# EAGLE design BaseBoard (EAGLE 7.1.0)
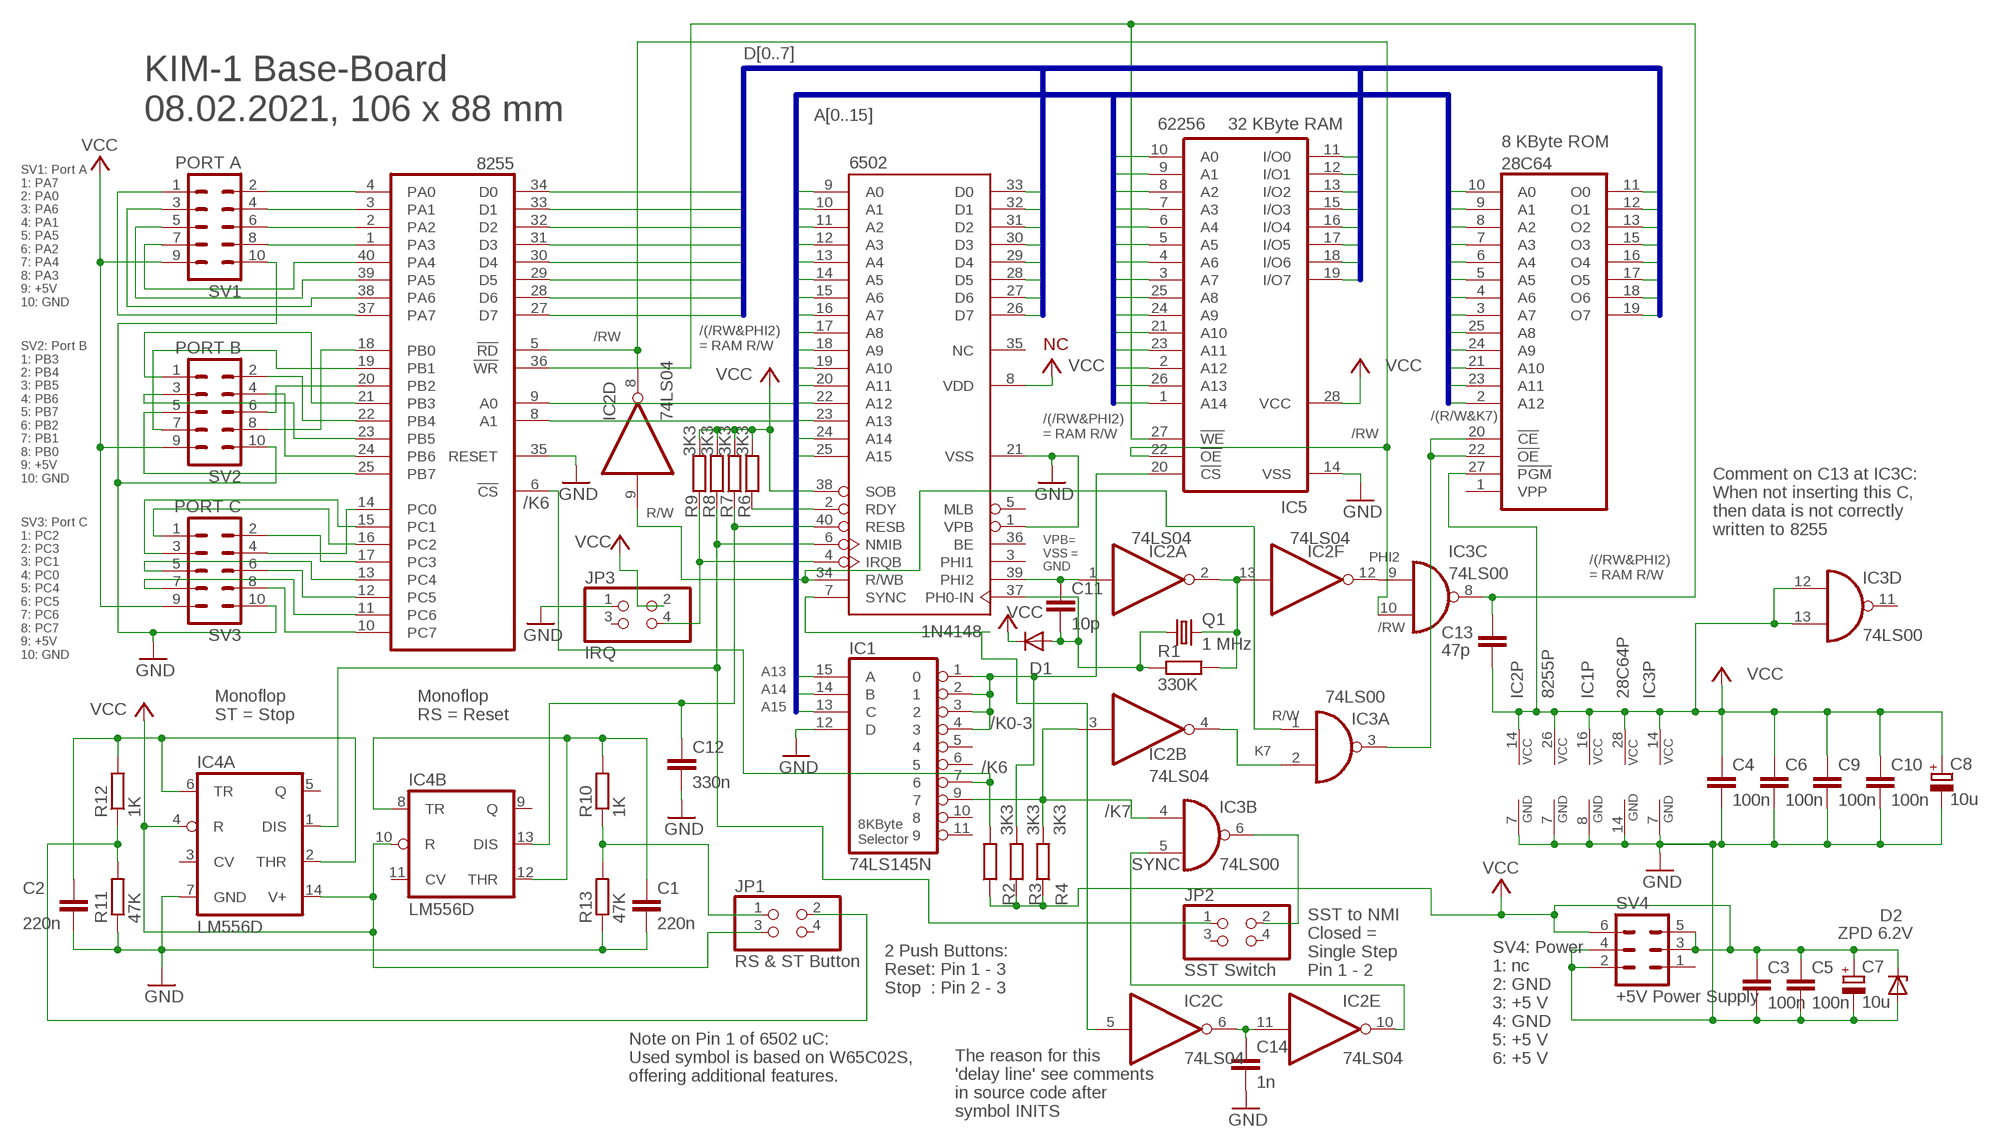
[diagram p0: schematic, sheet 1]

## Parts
28C64  2764  [DIL28]
6502  W65C02SP  [DIP-40]
8255  82C55A  [DIL40]
C1  220n  C-EUC1206  [C1206]
C2  220n  C-EUC1206  [C1206]
C3  100n  C-EUC1206  [C1206]
C4  100n  C-EUC1206  [C1206]
C5  100n  C-EUC1206  [C1206]
C6  100n  C-EUC1206  [C1206]
C7  10u  CPOL-EUE2.5-5  [E2,5-5]
C8  10u  CPOL-EUE2.5-5  [E2,5-5]
C9  100n  C-EUC1206  [C1206]
C10  100n  C-EUC1206  [C1206]
C11  10p  C-EUC1206  [C1206]
C12  330n  C-EUC1206  [C1206]
C13  47p  C-EUC1206  [C1206]
C14  1n  C-EUC1206  [C1206]
D1  1N4148  1N4148DO35-7  [DO35-7]
D2  ZPD 6.2V  ZPD  [DO35Z10]
IC1  74LS145N  [DIL16]
IC2  74LS04  74S04N  [DIL14]
IC3  74LS00  74ALS00N  [DIL14]
IC4  LM556D  [SO14]
IC5  62256  62256P  [DIL28-6]
JP1  RS & ST Button  PINHD-2X2  [2X02]
JP2  SST Switch  PINHD-2X2  [2X02]
JP3  IRQ  PINHD-2X2  [2X02]
Q1  1 MHz  CRYSTALHC18U-V  [HC18U-V]
R1  330K  R-EU_R1206  [R1206]
R2  3K3  R-EU_R1206  [R1206]
R3  3K3  R-EU_R1206  [R1206]
R4  3K3  R-EU_R1206  [R1206]
R6  3K3  R-EU_R1206  [R1206]
R7  3K3  R-EU_R1206  [R1206]
R8  3K3  R-EU_R1206  [R1206]
R9  3K3  R-EU_R1206  [R1206]
R10  1K  R-EU_R1206  [R1206]
R11  47K  R-EU_R1206  [R1206]
R12  1K  R-EU_R1206  [R1206]
R13  47K  R-EU_R1206  [R1206]
SV1  PORT A  ML10  [ML10]
SV2  PORT B  ML10  [ML10]
SV3  PORT C  ML10  [ML10]
SV4  +5V Power Supply  ML6  [ML6]

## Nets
A0: 28C64.10(A0) 6502.9(A0) 8255.9(A0) IC5.10(A0)
A1: 28C64.9(A1) 6502.10(A1) 8255.8(A1) IC5.9(A1)
A2: 28C64.8(A2) 6502.11(A2) IC5.8(A2)
A3: 28C64.7(A3) 6502.12(A3) IC5.7(A3)
A4: 28C64.6(A4) 6502.13(A4) IC5.6(A4)
A5: 28C64.5(A5) 6502.14(A5) IC5.5(A5)
A6: 28C64.4(A6) 6502.15(A6) IC5.4(A6)
A7: 28C64.3(A7) 6502.16(A7) IC5.3(A7)
A8: 28C64.25(A8) 6502.17(A8) IC5.25(A8)
A9: 28C64.24(A9) 6502.18(A9) IC5.24(A9)
A10: 28C64.21(A10) 6502.19(A10) IC5.21(A10)
A11: 28C64.23(A11) 6502.20(A11) IC5.23(A11)
A12: 28C64.2(A12) 6502.22(A12) IC5.2(A12)
A13: 6502.23(A13) IC1.15(A) IC5.26(A13)
A14: 6502.24(A14) IC1.14(B) IC5.1(A14)
A15: 6502.25(A15) IC1.13(C)
D0: 28C64.11(O0) 6502.33(D0) 8255.34(D0) IC5.11(I/O0)
D1: 28C64.12(O1) 6502.32(D1) 8255.33(D1) IC5.12(I/O1)
D2: 28C64.13(O2) 6502.31(D2) 8255.32(D2) IC5.13(I/O2)
D3: 28C64.15(O3) 6502.30(D3) 8255.31(D3) IC5.15(I/O3)
D4: 28C64.16(O4) 6502.29(D4) 8255.30(D4) IC5.16(I/O4)
D5: 28C64.17(O5) 6502.28(D5) 8255.29(D5) IC5.17(I/O5)
D6: 28C64.18(O6) 6502.27(D6) 8255.28(D6) IC5.18(I/O6)
D7: 28C64.19(O7) 6502.26(D7) 8255.27(D7) IC5.19(I/O7)
GND: 28C64.14(GND) 6502.1(VPB) 6502.21(VSS) 8255.7(GND) 8255.35(RESET) C1.2 C2.2 C3.2 C4.2 C5.2 C6.2 C7.- C8.- C9.2 C10.2 C12.2 C14.2 D2.A IC1.8(GND) IC1.12(D) IC2.7(P:GND) IC3.7(P:GND) IC4.7(A:GND) IC5.14(VSS) JP3.1 R11.1 R13.1 SV1.10 SV2.10 SV3.10 SV4.2 SV4.4
N$1: 8255.4(PA0) SV1.2
N$2: 8255.38(PA6) SV1.3
N$3: 8255.3(PA1) SV1.4
N$4: 8255.37(PA7) SV1.1
N$5: 8255.39(PA5) SV1.5
N$6: 8255.2(PA2) SV1.6
N$7: 8255.40(PA4) SV1.7
N$8: 8255.1(PA3) SV1.8
N$9: 6502.7(SYNC) IC2.5(C:I)
N$10: 8255.25(PB7) SV2.5
N$11: 8255.17(PC3) SV3.2
N$12: 8255.16(PC2) SV3.1
N$13: 8255.15(PC1) SV3.3
N$14: 8255.14(PC0) SV3.4
N$15: 8255.13(PC4) SV3.5
N$16: 8255.12(PC5) SV3.6
N$17: 8255.11(PC6) SV3.7
N$18: 8255.10(PC7) SV3.8
N$19: 8255.24(PB6) SV2.4
N$20: 8255.23(PB5) SV2.3
N$21: 8255.22(PB4) SV2.2
N$22: 8255.20(PB2) SV2.6
N$23: 8255.21(PB3) SV2.1
N$24: 8255.19(PB1) SV2.7
N$25: 8255.18(PB0) SV2.8
N$26: IC1.1 IC1.2 IC1.3 IC1.4 IC5.20(!CS) R3.2
N$27: IC1.9 IC2.3(B:I) IC3.4(B:I0) R4.2
N$28: 6502.39(PHI2) C11.1 IC2.1(A:I)
N$29: IC2.2(A:O) IC2.13(F:I) Q1.2 R1.2
N$30: 6502.37(PH0-IN) C11.2 D1.A Q1.1 R1.1
N$31: 8255.5(!RD) IC2.8(D:O) IC3.10(C:I1) IC5.22(!OE)
N$33: 8255.6(!CS) IC1.7 R2.2
N$34: IC2.4(B:O) IC3.2(A:I1)
N$35: 6502.34(R/WB) IC2.9(D:I) IC3.1(A:I0)
N$36: 6502.2(RDY) R6.1
N$37: 28C64.20(!CE) 28C64.22(!OE) IC3.3(A:O)
N$39: 6502.6(NMIB) IC4.1(A:DIS) JP2.1 R8.1
N$40: 6502.4(IRQB) JP3.4 R9.1
N$41: C2.1 IC4.2(A:THR) IC4.6(A:TR) R12.2
N$42: C1.1 IC4.8(B:TR) IC4.12(B:THR) R10.2
N$43: IC3.6(B:O) JP2.2
N$44: JP1.1 R10.1 R13.2
N$46: JP1.2 R11.2 R12.1
N$47: 6502.40(RESB) C12.1 IC4.13(B:DIS) R7.1
N$49: IC2.12(F:O) IC3.9(C:I0)
N$50: 8255.36(!WR) C13.1 IC3.8(C:O) IC5.27(!WE)
N$51: C14.1 IC2.6(C:O) IC2.11(E:I)
N$52: IC2.10(E:O) IC3.5(B:I1)
VCC: 28C64.27(!PGM) 28C64.28(VCC) 6502.8(VDD) 6502.38(SOB) 8255.26(VCC) C3.1 C4.1 C5.1 C6.1 C7.+ C8.+ C9.1 C10.1 C13.2 D1.C D2.C IC1.16(VCC) IC2.14(P:VCC) IC3.12(D:I0) IC3.13(D:I1) IC3.14(P:VCC) IC4.4(A:R) IC4.10(B:R) IC4.14(A:V+) IC5.28(VCC) JP1.3 JP3.2 R2.1 R3.1 R4.1 R6.2 R7.2 R8.2 R9.2 SV1.9 SV2.9 SV3.9 SV4.3 SV4.5 SV4.6
Unconnected: 28C64.1(VPP) 6502.3(PHI1) 6502.5(MLB) 6502.35(NC) 6502.36(BE) IC1.5 IC1.6 IC1.10 IC1.11 IC3.11(D:O) IC4.3(A:CV) IC4.5(A:Q) IC4.9(B:Q) IC4.11(B:CV) JP1.4 JP2.3 JP2.4 JP3.3 SV4.1

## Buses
A[0..15]
D[0..7]

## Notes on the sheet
- KIM-1 Base-Board
  08.02.2021, 106 x 88 mm
- 32 KByte RAM
- 8 KByte ROM
- SV1: Port A
  1: PA7
  2: PA0
  3: PA6
  4: PA1
  5: PA5
  6: PA2
  7: PA4
  8: PA3
  9: +5V
  10: GND
- /RW
- /(/RW&PHI2)
  = RAM R/W
- /(R/W&K7)
- /(/RW&PHI2)
  = RAM R/W
- /RW
- SV2: Port B
  1: PB3
  2: PB4
  3: PB5
  4: PB6
  5: PB7
  6: PB2
  7: PB1
  8: PB0
  9: +5V
  10: GND
- /K6
- R/W
- Comment on C13 at IC3C:
  When not inserting this C,
  then data is not correctly
  written to 8255
- PHI2
- VPB=
  VSS =
  GND
- /(/RW&PHI2)
  = RAM R/W
- /RW
- SV3: Port C
  1: PC2
  2: PC3
  3: PC1
  4: PC0
  5: PC4
  6: PC5
  7: PC6
  8: PC7
  9: +5V
  10: GND
- A13
- A14
- A15
- Monoflop
  ST = Stop
- Monoflop
  RS = Reset
- R/W
- /K0-3
- K7
- /K6
- /K7
- 8KByte
  Selector
- SYNC
- SST to NMI
  Closed =
  Single Step
  Pin 1 - 2
- 2 Push Buttons:
  Reset: Pin 1 - 3
  Stop  : Pin 2 - 3
- SV4: Power
  1: nc
  2: GND
  3: +5 V
  4: GND
  5: +5 V
  6: +5 V
- Note on Pin 1 of 6502 uC:
  Used symbol is based on W65C02S,
  offering additional features.
- The reason for this
  'delay line' see comments
  in source code after
  symbol INITS

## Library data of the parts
28C64 = memory:2764: MEMORY
6502 = 65xxx:W65C02SP: Western Digital Version
8255 = micro-harris:82C55A: MICROCONTROLLER/MEMORY DEVICE; MF: INTERSIL; MPN: CP82C55A-5; OC_FARNELL: 1018158; OC_NEWARK: 06F3290
C1-C6 C9-C14 = rcl:C-EU: CAPACITOR, European symbol
C7 C8 = rcl:CPOL-EU: POLARIZED CAPACITOR, European symbol
D1 = diode:1N4148: DIODE
D2 = diode:ZPD: Z DIODE
IC1 = 74xx-eu:74*145: BCD to decimal DECODER/DRIVER
IC2 = 74xx-eu:74*04: Hex INVERTER
IC3 = 74xx-eu:74*00: Quad 2-input NAND gate
IC4 = linear3:*556: Dual TIMER
IC5 = memory-hitachi:62256P: MEMORY; OC_FARNELL: unknown; OC_NEWARK: unknown
JP1-JP3 = pinhead:PINHD-2X2: PIN HEADER
Q1 = crystal:CRYSTAL: CRYSTAL; OC_FARNELL: unknown; OC_NEWARK: unknown
R1-R4 R6-R13 = rcl:R-EU_: RESISTOR, European symbol
SV1-SV3 = con-harting-ml:ML10: HARTING; OC_FARNELL: unknown; OC_NEWARK: unknown
SV4 = con-harting-ml:ML6: HARTING; OC_FARNELL: unknown; OC_NEWARK: unknown

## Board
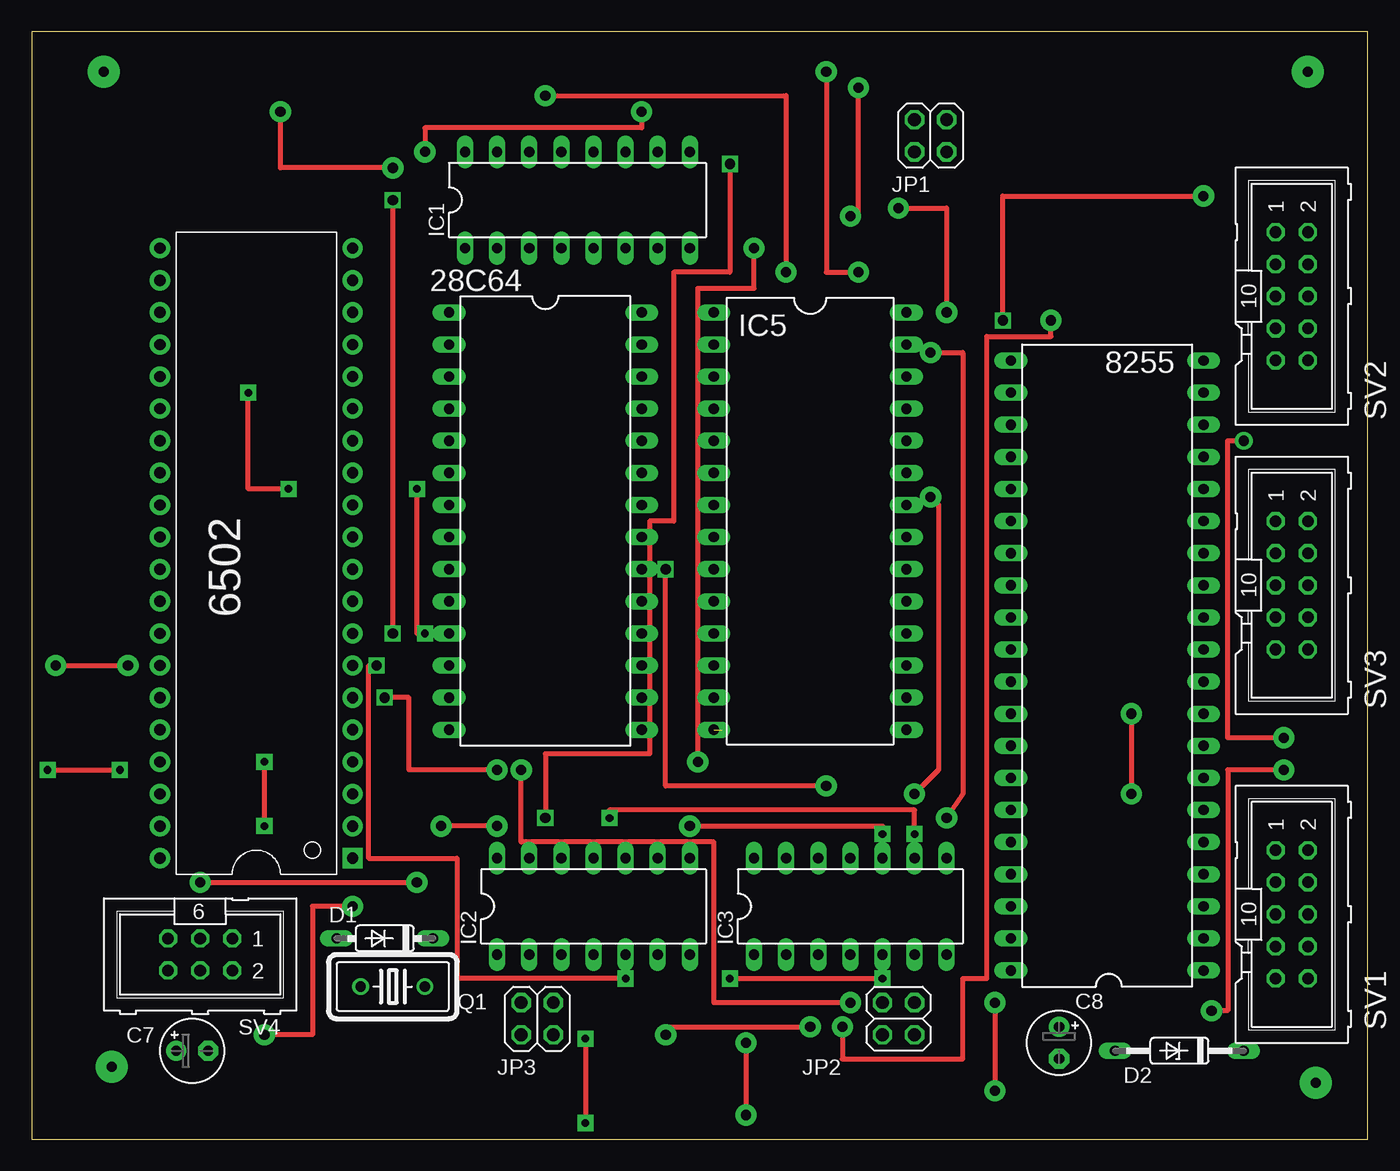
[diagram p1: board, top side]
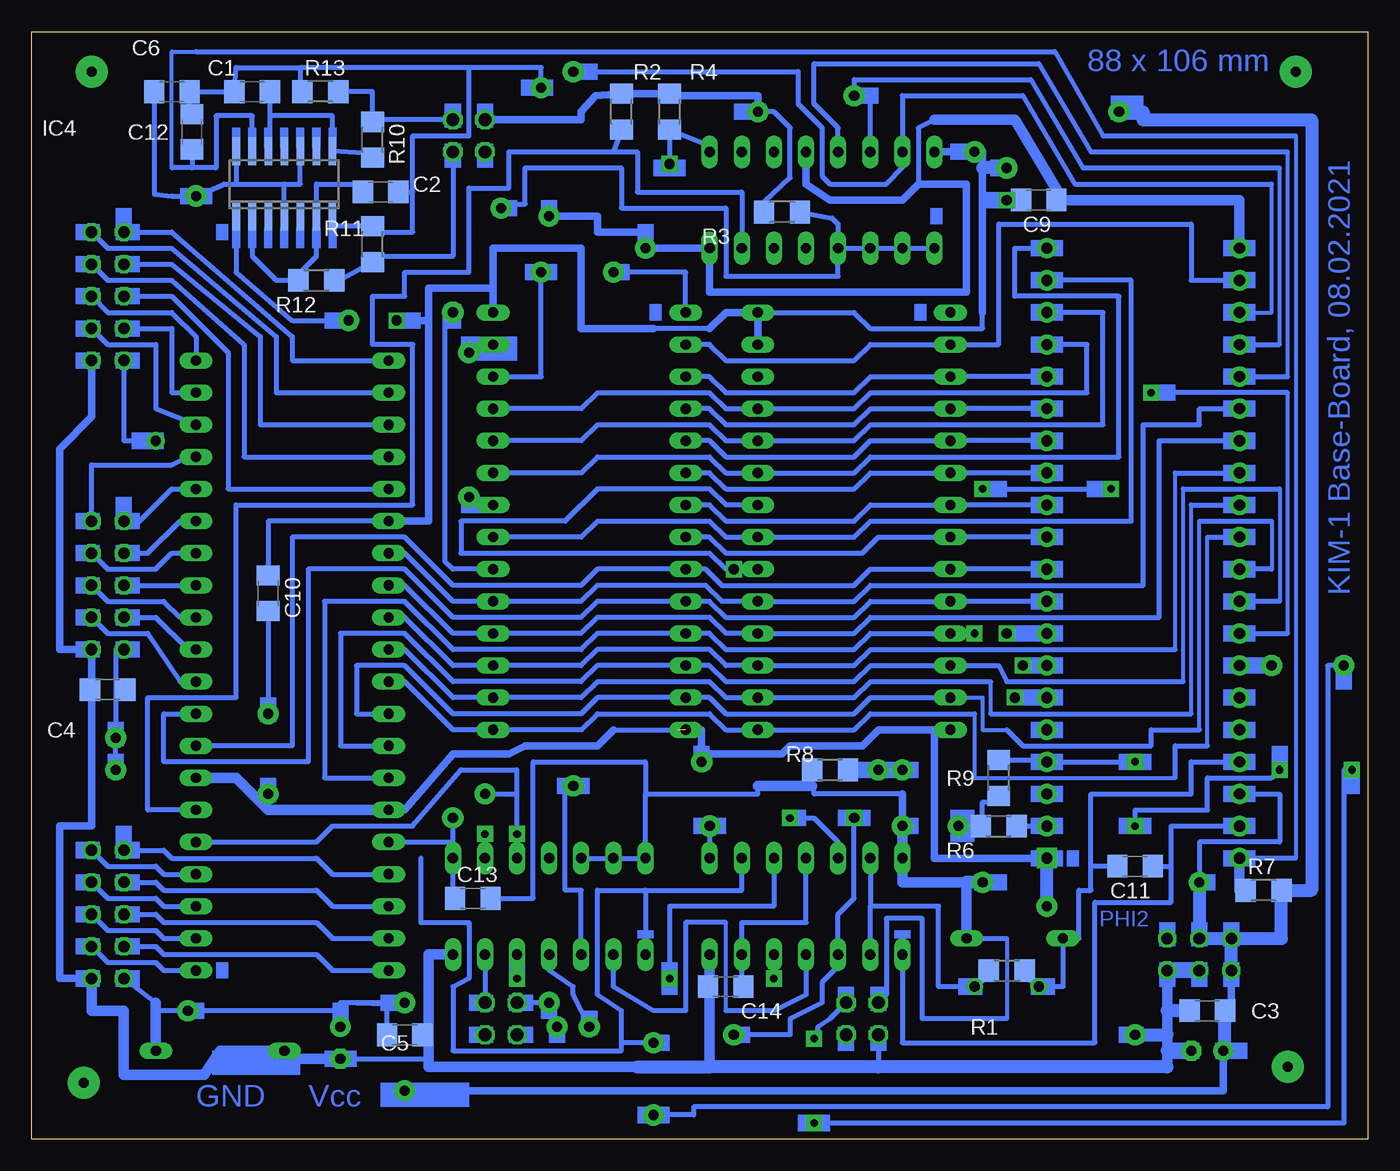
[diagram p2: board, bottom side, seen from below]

Size 105.72 x 87.62 mm. Coordinates in mm from the lower left corner, seen from the top.
Outline: 0,0 105.72,0 105.72,87.62 0,87.62 0,0
Copper layers (1*16): Top 0.035mm / dielectric 1.5mm / Bottom 0.035mm
Design rules "default": minimum track width 10mil, minimum drill 24mil, track to track 8mil, track to pad 8mil, pad to pad 8mil, via to via 8mil, smd to smd 8mil, copper to edge 40mil, drill to drill 8mil, minimum pad ring 10mil, minimum via ring 8mil, stop-mask expansion 4mil, vias tented up to drill 0mil, thermal gap 10mil

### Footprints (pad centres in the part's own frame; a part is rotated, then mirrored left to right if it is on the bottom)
DIL28 = drill 0.813 long: 1 -16.51,-7.62; 2 -13.97,-7.62; 3 -11.43,-7.62; 4 -8.89,-7.62; 5 -6.35,-7.62; 6 -3.81,-7.62; 7 -1.27,-7.62; 8 1.27,-7.62; 9 3.81,-7.62; 10 6.35,-7.62; 11 8.89,-7.62; 12 11.43,-7.62; 13 13.97,-7.62; 14 16.51,-7.62; 15 16.51,7.62; 16 13.97,7.62; 17 11.43,7.62; 18 8.89,7.62; 19 6.35,7.62; 20 3.81,7.62; 21 1.27,7.62; 22 -1.27,7.62; 23 -3.81,7.62; 24 -6.35,7.62; 25 -8.89,7.62; 26 -11.43,7.62; 27 -13.97,7.62; 28 -16.51,7.62
DIP-40 = drill 0.889 pad 1.6 square: 1 -22.86,-7.62 | drill 0.889 pad 1.6: 2 -20.32,-7.62; 3 -17.78,-7.62; 4 -15.24,-7.62; 5 -12.7,-7.62; 6 -10.16,-7.62; 7 -7.62,-7.62; 8 -5.08,-7.62; 9 -2.54,-7.62; 10 0,-7.62; 11 2.54,-7.62; 12 5.08,-7.62; 13 7.62,-7.62; 14 10.16,-7.62; 15 12.7,-7.62; 16 15.24,-7.62; 17 17.78,-7.62; 18 20.32,-7.62; 19 22.86,-7.62; 20 25.4,-7.62; 21 25.4,7.62; 22 22.86,7.62; 23 20.32,7.62; 24 17.78,7.62; 25 15.24,7.62; 26 12.7,7.62; 27 10.16,7.62; 28 7.62,7.62; 29 5.08,7.62; 30 2.54,7.62; 31 0,7.62; 32 -2.54,7.62; 33 -5.08,7.62; 34 -7.62,7.62; 35 -10.16,7.62; 36 -12.7,7.62; 37 -15.24,7.62; 38 -17.78,7.62; 39 -20.32,7.62; 40 -22.86,7.62
DIL40 = drill 0.813 long: 1 -24.13,-7.62; 2 -21.59,-7.62; 3 -19.05,-7.62; 4 -16.51,-7.62; 5 -13.97,-7.62; 6 -11.43,-7.62; 7 -8.89,-7.62; 8 -6.35,-7.62; 9 -3.81,-7.62; 10 -1.27,-7.62; 11 1.27,-7.62; 12 3.81,-7.62; 13 6.35,-7.62; 14 8.89,-7.62; 15 11.43,-7.62; 16 13.97,-7.62; 17 16.51,-7.62; 18 19.05,-7.62; 19 21.59,-7.62; 20 24.13,-7.62; 21 24.13,7.62; 22 21.59,7.62; 23 19.05,7.62; 24 16.51,7.62; 25 13.97,7.62; 26 11.43,7.62; 27 8.89,7.62; 28 6.35,7.62; 29 3.81,7.62; 30 1.27,7.62; 31 -1.27,7.62; 32 -3.81,7.62; 33 -6.35,7.62; 34 -8.89,7.62; 35 -11.43,7.62; 36 -13.97,7.62; 37 -16.51,7.62; 38 -19.05,7.62; 39 -21.59,7.62; 40 -24.13,7.62
C1206 = smd 1.6 x 1.8: 1 -1.4,0; 2 1.4,0
E2,5-5 = drill 0.813 pad 1.6: + -1.27,0 | drill 0.813 pad 1.6 octagon: - 1.27,0
DO35-7 = drill 0.813 long: A 3.81,0; C -3.81,0
DO35Z10 = drill 0.813 long: A 5.08,0; C -5.08,0
DIL16 = drill 0.813 long: 1 -8.89,-3.81; 2 -6.35,-3.81; 3 -3.81,-3.81; 4 -1.27,-3.81; 5 1.27,-3.81; 6 3.81,-3.81; 7 6.35,-3.81; 8 8.89,-3.81; 9 8.89,3.81; 10 6.35,3.81; 11 3.81,3.81; 12 1.27,3.81; 13 -1.27,3.81; 14 -3.81,3.81; 15 -6.35,3.81; 16 -8.89,3.81
DIL14 = drill 0.813 long: 1 -7.62,-3.81; 2 -5.08,-3.81; 3 -2.54,-3.81; 4 0,-3.81; 5 2.54,-3.81; 6 5.08,-3.81; 7 7.62,-3.81; 8 7.62,3.81; 9 5.08,3.81; 10 2.54,3.81; 11 0,3.81; 12 -2.54,3.81; 13 -5.08,3.81; 14 -7.62,3.81
SO14 = smd 0.6 x 2.2: 1 -3.81,-2.6; 2 -2.54,-2.6; 3 -1.27,-2.6; 4 0,-2.6; 5 1.27,-2.6; 6 2.54,-2.6; 7 3.81,-2.6; 8 3.81,2.6; 9 2.54,2.6; 10 1.27,2.6; 11 0,2.6; 12 -1.27,2.6; 13 -2.54,2.6; 14 -3.81,2.6
DIL28-6 = drill 0.813 long: 1 -16.51,-7.62; 2 -13.97,-7.62; 3 -11.43,-7.62; 4 -8.89,-7.62; 5 -6.35,-7.62; 6 -3.81,-7.62; 7 -1.27,-7.62; 8 1.27,-7.62; 9 3.81,-7.62; 10 6.35,-7.62; 11 8.89,-7.62; 12 11.43,-7.62; 13 13.97,-7.62; 14 16.51,-7.62; 15 16.51,7.62; 16 13.97,7.62; 17 11.43,7.62; 18 8.89,7.62; 19 6.35,7.62; 20 3.81,7.62; 21 1.27,7.62; 22 -1.27,7.62; 23 -3.81,7.62; 24 -6.35,7.62; 25 -8.89,7.62; 26 -11.43,7.62; 27 -13.97,7.62; 28 -16.51,7.62
2X02 = drill 1.016 octagon: 1 -1.27,-1.27; 2 -1.27,1.27; 3 1.27,-1.27; 4 1.27,1.27
HC18U-V = drill 0.813: 1 -2.54,0; 2 2.54,0
R1206 = smd 1.6 x 1.803: 1 -1.422,0; 2 1.422,0
ML10 = drill 0.914 octagon: 1 -5.08,-1.27; 2 -5.08,1.27; 3 -2.54,-1.27; 4 -2.54,1.27; 5 0,-1.27; 6 0,1.27; 7 2.54,-1.27; 8 2.54,1.27; 9 5.08,-1.27; 10 5.08,1.27
ML6 = drill 0.914 octagon: 1 -2.54,-1.27; 2 -2.54,1.27; 3 0,-1.27; 4 0,1.27; 5 2.54,-1.27; 6 2.54,1.27

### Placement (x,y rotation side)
28C64  40.64,48.9 270 top
6502  17.78,45.09 90 top
8255  85.09,37.47 90 top
C1  88.27,82.87 180 bottom
C2  78.11,74.93 0 bottom
C3  12.7,10.16 180 bottom
C4  99.7,35.56 180 bottom
C5  76.2,8.26 0 bottom
C6  94.62,82.87 0 bottom
C7  12.7,6.99 0 top
C8  81.28,7.62 270 top
C9  26.04,74.29 0 bottom
C10  87,43.18 270 bottom
C11  18.41,21.59 180 bottom
C12  93.03,79.69 90 bottom
C13  70.8,19.05 0 bottom
C14  50.8,12.07 180 bottom
D1  27.94,15.88 180 top
D2  90.81,6.99 180 top
IC1  43.18,74.29 0 top
IC2  44.45,18.41 0 top
IC3  64.77,18.41 0 top
IC4  85.73,75.56 0 bottom
IC5  61.59,48.9 270 top
JP1  71.12,79.38 180 top
JP2  68.58,9.53 270 top
JP3  40.01,9.53 0 top
Q1  28.57,12.07 0 top
R1  28.57,13.34 180 bottom
R2  59.05,81.28 270 bottom
R3  46.36,73.34 0 bottom
R4  55.25,81.28 270 bottom
R6  29.21,24.77 180 bottom
R7  8.26,19.69 0 bottom
R8  42.55,29.21 180 bottom
R9  29.21,28.57 270 bottom
R10  78.74,79.06 270 bottom
R11  78.74,70.8 270 bottom
R12  83.19,67.94 180 bottom
R13  82.87,82.87 0 bottom
SV1  99.7,17.78 270 top
SV2  99.7,66.67 270 top
SV3  99.7,43.81 270 top
SV4  13.34,14.61 180 top

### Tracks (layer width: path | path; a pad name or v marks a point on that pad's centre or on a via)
A0
  Bottom 0.406: 6502.9 28C64.10 39.37,42.55 40.64,41.27 50.8,41.27 52.07,42.55 IC5.10 60.96,42.55 62.23,41.27 72.39,41.27 76.2,45.09 83.82,45.09 83.82,29.84 95.25,29.84 95.25,33.66 8255.9
A1
  Bottom 0.406: 6502.10 28C64.9 39.37,45.09 40.64,43.81 51.12,43.81 52.39,45.09 IC5.9 60.96,45.09 62.23,43.81 72.39,43.81 76.2,47.62 85.09,47.62 85.09,31.12 8255.8
A2
  Bottom 0.406: 6502.11 28C64.8 38.73,47.62 40.01,46.35 50.8,46.35 52.07,47.62 IC5.8
A3
  Bottom 0.406: 6502.12 28C64.7 39.37,50.16 40.64,48.9 50.8,48.9 52.07,50.16 IC5.7
A4
  Bottom 0.406: 6502.13 28C64.6 39.37,52.7 40.64,51.44 50.8,51.44 52.07,52.7 IC5.6
A5
  Bottom 0.406: 6502.14 28C64.5 39.37,55.24 40.64,53.98 50.8,53.98 52.07,55.24 IC5.5
A6
  Bottom 0.406: 6502.15 28C64.4 39.37,57.79 40.64,56.52 50.8,56.52 52.07,57.79 IC5.4
A7
  Bottom 0.406: 6502.16 28C64.3 39.37,60.33 40.64,59.05 50.8,59.05 52.07,60.33 IC5.3
A8
  Bottom 0.406: 6502.17 22.22,62.87 22.22,59.05 39.37,59.05 40.64,57.79 28C64.25 50.8,57.79 52.07,59.05 60.96,59.05 62.23,57.79 IC5.25
A9
  Bottom 0.406: 6502.18 20.95,65.41 20.95,56.52 39.37,56.52 40.64,55.24 28C64.24 50.8,55.24 52.07,56.52 60.96,56.52 62.23,55.24 IC5.24
A10
  Bottom 0.406: 6502.19 18.73,67.94 18.73,48.9 39.37,48.9 40.64,47.62 28C64.21 50.8,47.62 52.07,48.9 60.96,48.9 62.23,47.62 IC5.21
A11
  Bottom 0.406: 6502.20 27.94,70.49 27.94,66.67 19.68,66.67 19.68,53.98 39.37,53.98 40.64,52.7 28C64.23 50.8,52.7 52.07,53.98 60.96,53.98 62.23,52.7 IC5.23
A12
  Bottom 0.406: 6502.22 13.97,67.94 13.97,72.39 29.21,72.39 29.21,62.87 28C64.2 39.37,62.87 40.64,61.59 50.8,61.59 52.07,62.87 IC5.2
A13  (via drill 0.8 pad 1.68)
  Top 0.406: v62.87,84.46 62.87,68.58 v65.41,68.58
  Bottom 0.305: 6502.23 7.62,65.41 7.62,75.56
  Bottom 0.406: 7.62,75.56 23.18,75.56 27.3,82.55 36.83,82.55 IC1.15 36.83,76.84 38.1,75.56 42.55,75.56 43.18,76.2 43.18,80.01 45.09,81.91 45.09,84.46 v62.87,84.46 | IC5.26 65.41,60.33 v65.41,68.58
A14  (via drill 0.8 pad 1.68)
  Top 0.406: v40.64,82.55 59.69,82.55 v59.69,68.58
  Bottom 0.305: 6.98,62.87 6.98,76.84
  Bottom 0.406: 6502.24 6.98,62.87 | IC1.14 39.37,82.55 v40.64,82.55 40.64,83.82 26.67,83.82 22.54,76.84 6.98,76.84 | IC5.1 53.98,68.58 v59.69,68.58
A15
  Bottom 0.305: 6.35,60.33 6.35,78.1
  Bottom 0.406: 6502.25 6.35,60.33 | IC1.13 41.91,80.01 43.82,81.91 43.82,85.09 26.04,85.09 21.91,78.1 6.35,78.1
D0  (via drill 0.6 pad 1.27)
  Top 0.406: v31.11,40.01 30.48,40.01 v30.48,51.44 | v20.32,51.44 17.14,51.44 v17.14,59.05
  Bottom 0.305: 6.35,40.01 6.35,59.05
  Bottom 0.406: 8255.34 82.55,28.57 82.55,42.55 76.2,42.55 72.39,38.73 62.23,38.73 60.96,40.01 IC5.11 52.07,40.01 50.8,38.73 40.64,38.73 39.37,40.01 28C64.11 v31.11,40.01 | 6502.33 6.35,40.01 | 6.35,59.05 v17.14,59.05 | v30.48,51.44 v20.32,51.44
D1
  Bottom 0.305: 14.61,36.2 14.61,51.44 | 6.98,51.44 6.98,42.55
  Bottom 0.406: 14.61,36.2 28.57,36.2 29.21,37.47 28C64.12 39.37,37.47 40.64,36.2 50.8,36.2 52.07,37.47 IC5.12 60.96,37.47 62.23,36.2 72.39,36.2 76.2,40.01 81.28,40.01 81.28,31.12 8255.33 | 14.61,51.44 6.98,51.44 | 6.98,42.55 6502.32
D2
  Bottom 0.305: 28C64.13 30.48,34.92 30.48,32.39 28.57,32.39 | 13.34,32.39 13.34,48.9 | 7.62,48.9 7.62,45.09
  Bottom 0.406: 28C64.13 39.37,34.92 40.64,33.66 50.8,33.66 52.07,34.92 IC5.13 60.96,34.92 62.23,33.66 72.39,33.66 76.2,37.47 80.01,37.47 80.01,33.66 8255.32 | 28.57,32.39 27.3,31.12 17.14,31.12 17.14,32.39 13.34,32.39 | 13.34,48.9 7.62,48.9 | 7.62,45.09 6502.31
D3
  Bottom 0.305: 31.11,33.66 31.11,28.57 15.24,28.57 | 12.7,31.12 12.7,47.62
  Bottom 0.406: 8255.31 76.2,36.2 72.39,32.39 IC5.15 62.23,32.39 60.96,33.66 52.07,33.66 50.8,32.39 28C64.15 40.64,32.39 39.37,33.66 31.11,33.66 | 15.24,28.57 15.24,31.12 12.7,31.12 | 12.7,47.62 6502.30
D4
  Bottom 0.305: 29.84,36.2 29.84,33.66 | 13.97,33.66 13.97,50.16
  Bottom 0.406: 8255.30 76.2,38.73 72.39,34.92 IC5.16 62.23,34.92 60.96,36.2 52.07,36.2 50.8,34.92 28C64.16 40.64,34.92 39.37,36.2 29.84,36.2 | 29.84,33.66 13.97,33.66 | 13.97,50.16 6502.29
D5
  Bottom 0.305: 15.24,38.73 15.24,52.7
  Bottom 0.406: 8255.29 76.2,41.27 72.39,37.47 IC5.17 62.23,37.47 60.96,38.73 52.07,38.73 50.8,37.47 28C64.17 40.64,37.47 39.37,38.73 15.24,38.73 | 15.24,52.7 6502.28
D6
  Bottom 0.406: 8255.28 76.2,43.81 72.39,40.01 IC5.18 62.23,40.01 60.96,41.27 52.07,41.27 50.8,40.01 28C64.18 40.64,40.01 39.37,41.27 16.51,41.27 16.51,55.24 6502.27
D7
  Bottom 0.406: 8255.27 76.2,46.35 72.39,42.55 IC5.19 62.23,42.55 60.96,43.81 52.39,43.81 51.12,42.55 28C64.19 40.64,42.55 39.37,43.81 17.78,43.81 17.78,56.52 13.34,56.52 13.34,57.79 6502.26
GND  (via drill 0.8 pad 1.68)  (1 unrouted)
  Top 0.406: v52.71,29.84 52.71,67.31 57.15,67.31 v57.15,70.49 | v64.77,73.03 65.41,73.03 v65.41,83.19 | v25.4,18.41 22.22,18.41 22.22,8.26 v18.41,8.26 | v87,33.66 v87,27.3
  Bottom 0.406: 34.29,32.39 28C64.14 | 34.29,80.65 35.56,80.01 35.56,75.56 | 8255.35 76.2,26.04 | 84.45,84.77 89.53,84.77 89.67,83.06 C1.2 C6.2 93.22,81.09 C12.2 | 84.45,84.77 84.45,82.4 R13.1 | IC4.7 81.92,72.22 R11.1 78.74,71.75 75.56,71.75 75.56,74.93 | 75.56,74.93 75.56,79.38 71.12,79.38 71.12,84.77 | 71.12,84.77 84.45,84.77 | C2.2 75.56,74.93 | v65.41,83.19 65.41,84.77 71.12,84.77 | C5.2 74.3,8.26 | C8.- 74.3,6.35 | C4.2 100.97,35.56 | 59.69,32.39 54.61,32.39 | C9.2 24.3,74.29 24.3,74.57 | C10.2 v87,33.66 | v87,27.3 87,26.04 | JP3.1 38.73,5.71 | C14.2 52.07,12.07 IC2.7
  Bottom 0.61: 28C64.14 38.73,32.39 40.01,31.12 45.72,31.12 46.36,30.48 52.71,30.48 | 52.71,30.48 52.71,32.39 IC5.14 | 76.2,26.04 72.39,30.48 67.95,30.48 66.67,31.12 60.96,31.12 59.69,32.39 | 6502.1 34.29,22.23 34.29,32.39 | v52.71,29.84 52.71,30.48 | IC1.12 44.45,75.56 42.55,74.29 36.83,74.29 35.56,75.56 31.75,75.56 31.75,66.99 52.07,66.99 IC1.8 v57.15,70.49 57.15,71.75 60.96,71.75 60.96,73.03 v64.77,73.03 | SV2.10 100.97,57.15 103.5,54.61 103.5,38.73 SV3.10 100.97,35.56 100.97,24.77 103.5,24.77 103.5,12.7 SV1.10
  Bottom 0.813: 8255.7 89.53,28.57 87,26.04 8255.35 | 6502.21 10.16,74.29 24.13,74.29 24.3,74.57 27.94,80.65 34.29,80.65 | IC3.7 74.3,14.61 74.3,8.26 74.3,6.35 74.3,5.71 57.79,5.71 | 52.07,5.71 IC2.7 | SV4.2 15.88,10.16 15.88,8.26 15.88,6.99 15.88,5.71 | C8.- 85.73,6.35 D2.A 90.81,6.99 92.08,5.08 98.42,5.08 98.42,10.16 100.97,10.16 SV1.10
  Bottom 1.016: 57.79,5.71 52.07,5.71 38.73,5.71 15.88,5.71 | C3.2 15.88,10.16 | v18.41,8.26 15.88,8.26 | v25.4,18.41 6502.1 | C7.- 15.88,6.99
  Bottom 1.27: SV4.4 SV4.2
N$1
  Bottom 0.406: SV1.2 99.7,21.59 95.89,21.59 95.25,20.96 8255.4
N$2
  Bottom 0.406: SV1.3 95.89,20.32 95.25,19.69 83.19,19.69 81.92,18.41 8255.38
N$3
  Bottom 0.406: SV1.4 99.7,19.05 95.89,19.05 95.25,18.41 8255.3
N$4
  Bottom 0.406: SV1.1 95.25,22.86 94.62,22.23 83.19,22.23 81.92,20.96 8255.37
N$5
  Bottom 0.406: SV1.5 95.89,17.78 95.25,17.14 83.19,17.14 81.92,15.88 8255.39
N$6
  Bottom 0.406: SV1.6 99.7,16.51 95.89,16.51 95.25,15.88 8255.2
N$7
  Bottom 0.406: SV1.7 95.89,15.24 95.25,14.61 83.19,14.61 81.92,13.34 8255.40
N$8
  Bottom 0.406: SV1.8 99.7,13.97 95.89,13.97 95.25,13.34 8255.1
N$9  (via drill 0.6 pad 1.27, 0.8 pad 1.27)
  Top 0.406: v27.3,37.47 26.67,37.47 26.67,22.23 33.66,22.23 33.66,12.7 v46.99,12.7
  Bottom 0.406: v27.3,37.47 6502.7 | IC2.5 v46.99,12.7
N$10
  Bottom 0.406: SV2.5 94.62,66.67 90.17,62.23 90.17,51.44 8255.25
N$11
  Bottom 0.406: SV3.2 100.97,53.34 94.62,53.34 93.34,53.98 8255.17
N$12
  Bottom 0.406: SV3.1 97.16,48.9 94.62,51.44 8255.16
N$13
  Bottom 0.406: SV3.3 96.52,46.35 93.98,48.9 8255.15
N$14
  Bottom 0.406: SV3.4 99.7,45.09 95.89,45.09 94.62,46.35 8255.14
N$15
  Bottom 0.406: SV3.5 8255.13
N$16
  Bottom 0.406: SV3.6 99.7,42.55 95.25,42.55 93.98,41.27 8255.12
N$17
  Bottom 0.406: SV3.7 95.89,41.27 93.34,38.73 8255.11
N$18
  Bottom 0.406: SV3.8 99.7,40.01 96.52,40.01 93.98,36.2 8255.10
N$19
  Bottom 0.406: SV2.4 99.7,67.94 94.62,67.94 88.9,62.87 88.9,53.98 8255.24
N$20
  Bottom 0.406: SV2.3 94.62,69.22 87.63,63.5 87.63,56.52 8255.23
N$21
  Bottom 0.406: SV2.2 99.7,70.49 94.62,70.49 86.36,63.5 86.36,59.05 8255.22
N$22
  Bottom 0.406: SV2.6 99.7,65.41 94.62,65.41 92.71,63.5 8255.20
N$23
  Bottom 0.406: SV2.1 94.62,71.75 85.09,63.5 85.09,61.59 8255.21
N$24
  Bottom 0.406: SV2.7 94.62,64.13 94.62,59.05 8255.19
N$25
  Bottom 0.406: SV2.8 99.7,62.87 95.89,62.87 95.89,57.79 8255.18
N$26  (via drill 0.8 pad 1.68)
  Top 0.406: v68.58,73.66 72.39,73.66 v72.39,65.41
  Bottom 0.406: v68.58,73.66 68.58,73.98 66.67,73.98 66.67,76.84 59.05,76.84 59.05,73.66 50.8,73.66 50.8,68.26 41.91,68.26 IC1.4 | IC1.4 IC1.3 IC1.2 IC1.1 34.14,70.64 34.29,70.64 | IC5.20 72.39,45.09 73.03,45.72 73.03,65.41 v72.39,65.41 | R3.2 42.39,72.87 41.91,72.39 IC1.4
N$27  (via drill 0.8 pad 1.27, 0.8 pad 1.68)
  Top 0.406: v50.16,8.26 50.16,8.89 v61.59,8.89 | v55.25,77.15 55.25,68.58 50.8,68.58 50.8,48.9 48.9,48.9 48.9,30.48 40.64,30.48 v40.64,25.4
  Bottom 0.406: v50.16,8.26 45.72,8.26 45.72,9.53 43.18,10.79 43.18,12.38 41.91,13.65 IC2.3 41.91,17.78 40.64,19.05 v40.64,25.4 | v61.59,8.89 62.87,11.43 62.87,12.07 64.77,13.34 IC3.4 | IC1.9 52.07,78.59 R4.2 v55.25,77.15
N$28
  Bottom 0.406: IC2.1 36.83,7.62 21.59,7.62 21.59,18.73 15.56,18.73 15.56,21.59 | 15.56,21.59 15.56,24.77 6502.39 | C11.1 15.56,21.59
N$29
  Bottom 0.406: R1.2 30,12.85 Q1.2 33.97,12.07 33.97,18.41 39.37,18.41 | IC2.2 39.37,18.41 | IC2.13 39.37,18.41
N$30
  Bottom 0.406: 21.91,21.59 21.91,19.69 22.86,19.69 22.86,15.88 D1.A 24.13,12.07 Q1.1 27.15,12.85 R1.1 | 21.91,21.59 21.91,27.3 13.97,27.3 13.97,29.84 6502.37 | C11.2 21.91,21.59
N$31  (via drill 0.6 pad 1.27, 0.8 pad 1.68)
  Top 0.406: v52.07,24.77 67.31,24.77 v67.31,24.13 | v69.85,27.3 71.75,29.21 71.75,50.16 v71.12,50.8
  Bottom 0.406: 8255.5 83.19,23.5 81.92,24.77 75.56,24.77 71.75,29.21 67.31,29.21 67.31,27.3 | IC3.10 v67.31,24.13 67.31,27.3 | v52.07,24.77 IC2.8 | v69.85,27.3 67.31,27.3 | IC5.22 70.48,50.16 v71.12,50.8
N$32  (via drill 0.8 pad 2.54)
  other vias: 5.71,84.46
N$33
  Bottom 0.406: 59.69,78.1 67.95,78.1 67.95,75.25 71.12,75.25 71.12,68.58 76.2,68.58 76.2,66.67 78.74,66.67 78.74,62.87 75.56,62.87 75.56,50.16 89.53,50.16 89.53,34.92 96.52,34.92 96.52,26.04 8255.6 | 59.69,78.1 57.79,78.1 57.79,74.93 49.53,74.93 IC1.7 | R2.2 59.69,78.1
N$34
  Bottom 0.305: 50.8,10.16 50.8,17.14
  Bottom 0.406: IC2.4 44.45,11.43 46.99,10.16 50.8,10.16 | 50.8,17.14 53.98,17.14 53.98,10.16 56.52,10.16 59.69,12.07 IC3.2
N$35  (via drill 0.8 pad 1.68)
  Top 0.406: v56.52,7.62 v56.52,1.91 | v1.91,37.47 v7.62,37.47
  Bottom 0.406: 74.93,22.23 74.93,17.14 71.12,17.14 71.12,12.7 72.39,12.07 72.39,6.99 59.05,6.99 59.05,7.62 | 59.05,7.62 59.05,10.16 60.96,11.43 60.96,19.69 57.15,19.69 | 57.15,19.69 IC3.1 | 57.15,19.69 49.53,19.69 IC2.9 | v7.62,37.47 6502.34 | v56.52,7.62 59.05,7.62 | v1.91,37.47 3.17,37.47 3.17,2.54 53.34,2.54 53.34,1.91 v56.52,1.91
N$36
  Bottom 0.406: R6.1 6502.2
N$37  (via drill 0.8 pad 1.27, 0.8 pad 1.68)
  Top 0.406: v62.87,27.94 50.16,27.94 v50.16,45.09
  Bottom 0.406: 28C64.20 v50.16,45.09 50.8,45.09 52.07,46.35 71.75,46.35 71.75,48.9 63.5,48.9 60.96,51.44 52.07,51.44 50.8,50.16 28C64.22 | IC3.3 62.23,19.69 63.5,19.69 63.5,27.3 v62.87,27.94
N$38  (via drill 0.8 pad 2.54)
  other vias: 100.97,84.46
N$39  (via drill 0.8 pad 1.27, 0.8 pad 1.68)
  Top 0.406: v36.83,29.21 29.84,29.21 29.84,34.92 v27.94,34.92 | v64.77,10.79 53.98,10.79 53.98,23.5 38.73,23.5 v38.73,29.21 | v64.14,8.89 64.14,6.35 73.66,6.35 73.66,12.7 75.56,12.7 75.56,63.5 80.64,63.5 v80.64,64.77
  Bottom 0.406: 6502.6 v27.94,34.92 | JP2.1 v64.77,10.79 v64.14,8.89 | v36.83,29.21 v38.73,29.21 R8.1 | IC4.1 89.53,68.58 85.09,64.77 v80.64,64.77
N$40  (via drill 0.6 pad 1.27)
  Top 0.406: v18.41,29.84 v18.41,24.77 | v1.27,29.21 v6.98,29.21 | v43.82,7.94 v43.82,1.27
  Bottom 0.406: R9.1 25.55,30 6502.4 v18.41,29.84 | v18.41,24.77 18.41,26.04 12.7,26.04 12.7,28.57 7.62,28.57 v6.98,29.21 | v43.82,7.94 43.5,8.57 43.5,8.89 42.55,9.53 JP3.4 | v1.27,29.21 1.91,29.21 1.91,1.27 v43.82,1.27
N$41
  Bottom 0.406: 84.45,67.79 R12.2 | R12.2 84.61,68.43 83.19,69.85 IC4.6 83.19,75.56 80.01,75.56 80.01,74.93 C2.1 79.38,74.93 | IC4.2 88.27,69.85 86.36,67.94 R12.2
N$42
  Bottom 0.406: R10.2 78.84,77.95 IC4.8 | C1.1 86.87,80.96 | 86.87,80.96 86.87,80.2 IC4.12 | IC4.8 81.92,78.1 | IC4.8 81.92,80.96 86.87,80.96
N$43
  Bottom 0.406: IC3.6 JP2.2
N$44
  Bottom 0.406: R13.2 78.74,82.87 R10.1 78.74,80.65 JP1.1
N$45  (via drill 0.8 pad 2.54)
  other vias: 101.6,4.45
N$46
  Bottom 0.406: R12.1 81.61,67.79 R11.2 78.74,69.7 78.11,69.85 72.39,69.85 JP1.2
N$47
  Bottom 0.305: 94.62,76.84 94.62,86.04 92.71,86.04 | 5.71,79.38 5.71,22.23
  Bottom 0.406: IC4.13 88.27,80.96 91.12,80.96 91.12,76.84 93.03,76.84 | 93.03,76.84 94.62,76.84 | 92.71,86.04 24.76,86.04 20.95,79.38 5.71,79.38 | 10.01,22.38 6502.40 5.71,22.23 | C12.1 93.03,76.84
  Bottom 0.813: R7.1 10.16,19.69 6502.40
N$48  (via drill 0.8 pad 2.54)
  other vias: 6.35,5.71
N$49  (via drill 0.6 pad 1.27)
  Top 0.406: v69.85,24.13 69.85,26.04 45.72,26.04 v45.72,25.4
  Bottom 0.406: v45.72,25.4 43.82,25.4 41.91,23.5 IC2.12 | v69.85,24.13 IC3.9
N$50  (via drill 0.8 pad 1.68)
  Top 0.406: v71.12,62.23 73.66,62.23 73.66,27.3 v72.39,25.4
  Bottom 0.406: 72.39,23.5 IC3.8 72.39,19.05 C13.1 | 72.39,23.5 v72.39,25.4 | v71.12,62.23 70.48,62.23 69.85,62.87 IC5.27 | 8255.36 72.39,23.5
N$51
  Bottom 0.406: IC2.11 44.45,17.14 49.53,17.14 IC2.6 49.53,12.07 C14.1
N$52  (via drill 0.6 pad 1.27)
  Top 0.406: v55.25,12.7 v67.31,12.7
  Bottom 0.406: v67.31,12.7 IC3.5 | IC2.10 46.99,18.41 55.25,18.41 v55.25,12.7
VCC  (via drill 0.8 pad 1.27, 0.8 pad 1.42, 0.8 pad 1.68)
  Top 0.406: v36.83,24.77 v32.38,24.77 | v28.57,74.29 v28.57,40.01 | v76.84,64.77 76.84,74.61 v92.71,74.61 | v99.06,29.21 94.62,29.21 94.62,10.16 v93.34,10.16 | v99.06,31.75 94.62,31.75 94.62,55.24 v95.89,55.24 | v13.34,20.32 v30.48,20.32 | v48.26,81.28 48.26,80.01 31.11,80.01 v31.11,78.1 | v28.57,76.84 19.68,76.84 v19.68,81.28 | v76.2,10.79 v76.2,3.81
  Bottom 0.305: 28.57,15.88 28.57,9.53
  Bottom 0.406: v48.26,81.28 46.99,81.28 45.72,80.01 45.72,76.05 47.78,74.14 47.62,73.66 R3.1 | R9.2 28.57,26.67 30.48,26.67 30.48,24.77 R6.2 v32.38,24.77 | IC4.10 84.45,75.56 85.73,75.56 | IC4.14 89.53,75.56 | 89.53,75.56 85.73,75.56 | 30.48,74.29 v28.57,74.29 C9.1 | v28.57,40.01 6502.8 | 89.53,75.56 90.49,75.56 v92.71,74.61 94.62,74.61 96.02,74.74 C6.1 | IC3.12 IC3.13 IC3.14 57.15,27.3 | R8.2 43.97,27.94 43.82,27.94 43.82,27.3 36.83,27.3 | 48.26,27.94 48.26,27.3 57.15,27.3 | IC4.4 85.73,75.56 | SV1.9 95.89,10.79 95.89,10.16 v93.34,10.16 81.28,10.16 | v99.06,29.21 v99.06,31.75 99.06,35.56 | SV2.9 98.42,55.24 v95.89,55.24 | SV3.9 99.06,38.73 99.06,35.56 | v76.2,10.79 81.28,10.79 | 81.28,10.79 81.28,10.16 | C7.+ 11.3,6.99 | C3.1 11.3,10.66 | C5.1 77.6,10.66 81.28,10.79 | C8.+ 81.28,10.16 | C4.1 99.06,35.56 | 6502.38 6.98,27.3 6.98,23.5 13.34,23.5 v13.34,20.32 | 8255.26 87,48.9 C10.1 | 28C64.28 40.64,65.41 39.37,64.13 30.48,64.13 30.48,65.41 | 52.07,64.13 56.52,64.13 | D1.C 28.57,15.88 | 28.57,9.53 35.24,9.53 35.24,17.46 38.1,17.46 38.1,11.43 JP3.2 | C13.2 66.04,19.05 66.04,29.84 57.15,29.84 57.15,27.3
  Bottom 0.61: 52.07,64.13 50.8,65.41 28C64.28 28C64.27 | 8255.26 74.3,48.9 74.3,64.77 | 74.3,64.77 74.3,67.31 69.22,67.31 | IC1.16 v31.11,78.1 30.48,78.1 30.48,76.84 30.48,74.29 30.48,65.41 | v76.84,64.77 74.3,64.77 | 36.83,27.3 v36.83,24.77 | 11.3,10.66 10.79,10.66 SV4.6 | JP1.3 62.23,80.65 62.23,81.28 61.11,82.55 R2.1 R4.1 55.25,82.55 48.26,82.55 v48.26,81.28 | 69.22,67.31 IC5.28 | C7.+ 11.43,3.81 v76.2,3.81 | 69.22,67.31 69.22,70.49 62.23,70.49 62.23,64.13 56.52,64.13
  Bottom 0.813: D1.C 31.75,20.32 36.83,20.32 IC2.14 v36.83,24.77 | 48.26,27.94 43.97,27.94 | D2.C 95.89,10.79
  Bottom 1.016: 11.3,6.99 C3.1 | SV4.6 SV4.5 | SV4.5 SV4.3 v13.34,20.32 | SV4.5 6.83,15.88 R7.2 4.45,19.69 4.45,80.65 17.78,80.65 17.78,81.28 v19.68,81.28 | v30.48,20.32 31.75,20.32 | v28.57,76.84 30.48,76.84
(copper drawn outside any net)
  shapes: Bottom area x184

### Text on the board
Bottom: 88 x 106 mm | KIM-1 Base-Board, 08.02.2021 | PHI2 | Vcc | GND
